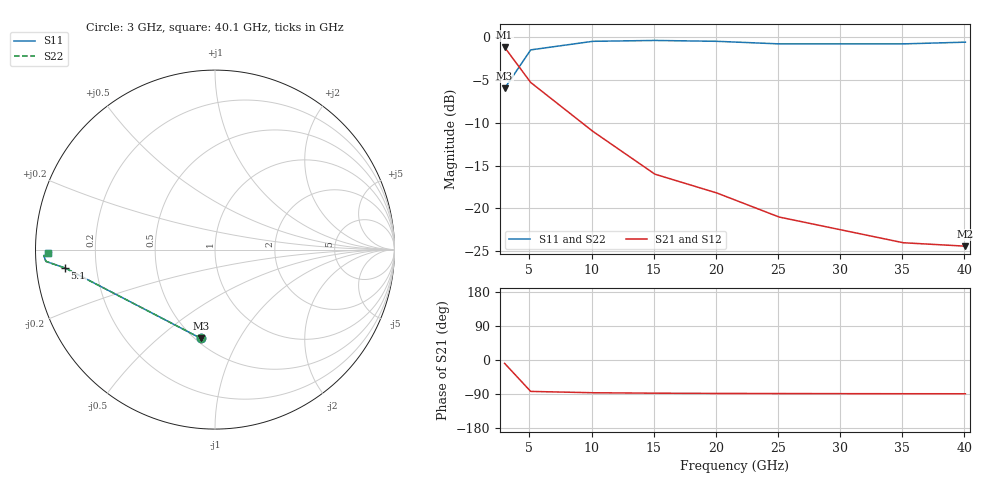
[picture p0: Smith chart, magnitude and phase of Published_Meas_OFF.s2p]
! Created Wed May 09 10:00:44 2001
# hz S db R 50
! SP2.SP
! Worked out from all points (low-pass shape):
!   9 points, 3 GHz to 40.1 GHz, reference 50 ohm
!   highest |S21| = -1.20 dB at 3 GHz (marker M1); lowest = -24.4 dB at 40.1 GHz (marker M2)
!   |S21| within 3 dB of the highest: start of sweep to 4.537 GHz
!   lowest |S11| = -6.0 dB at 3 GHz (marker M3), VSWR 3.01, Z = 26.6 - j35.2 ohm
!   |S11| at or under -10 dB: nowhere
!   |S22| runs from -6.0 to -0.4 dB; largest |S21 - S12| = 0
!   S11 on the Smith chart (normalised r, x): 3 GHz: 0.53, -0.70; 5.1 GHz: 0.09, -0.06; 40.1 GHz: 0.03, -0.01
3e9  -6.00 -98.9  -1.20 -8.9  -1.20 -8.9  -6.00 -98.9
5.1e9  -1.50 -173.0  -5.30 -82.9  -5.30 -82.9  -1.50 -173.0
1.01e10  -0.50 -176.0  -11.00 -86.4  -11.00 -86.4  -0.50 -176.0
1.51e10  -0.40 -178.0  -16.00 -87.6  -16.00 -87.6  -0.40 -178.0
2.01e10  -0.50 -178.0  -18.20 -88.2  -18.20 -88.2  -0.50 -178.0
2.51e10  -0.80 -179.0  -21.00 -88.5  -21.00 -88.5  -0.80 -179.0
3.01e10  -0.80 -179.0  -22.50 -88.8  -22.50 -88.8  -0.80 -179.0
3.51e10  -0.80 -179.0  -24.00 -89.0  -24.00 -89.0  -0.80 -179.0
4.01e10  -0.60 -179.0  -24.40 -89.1  -24.40 -89.1  -0.60 -179.0
